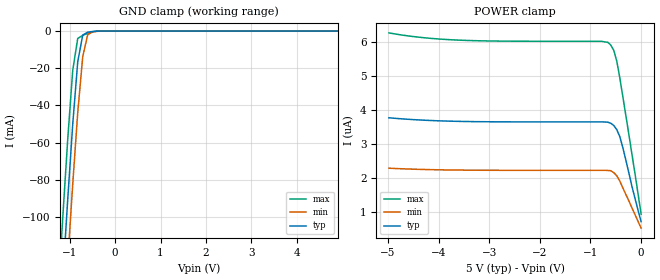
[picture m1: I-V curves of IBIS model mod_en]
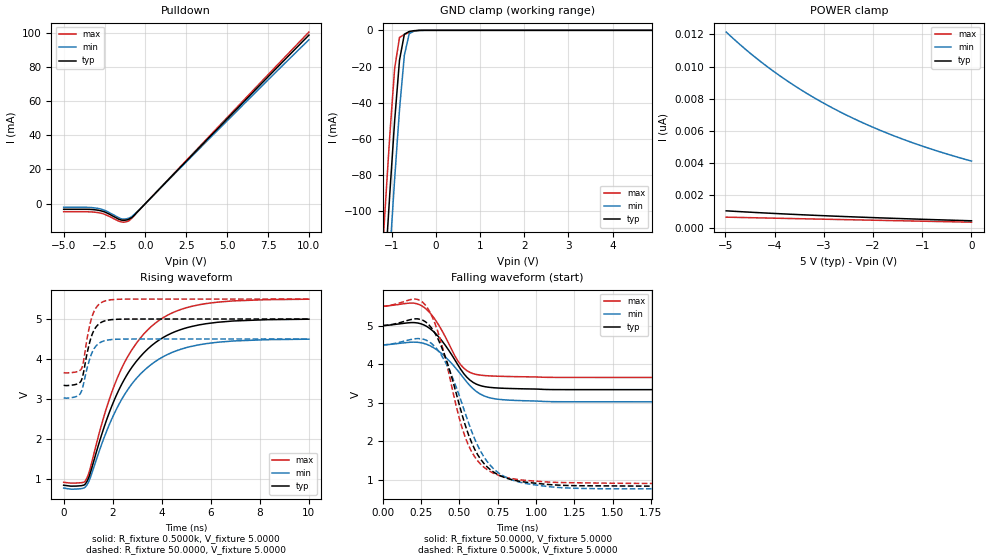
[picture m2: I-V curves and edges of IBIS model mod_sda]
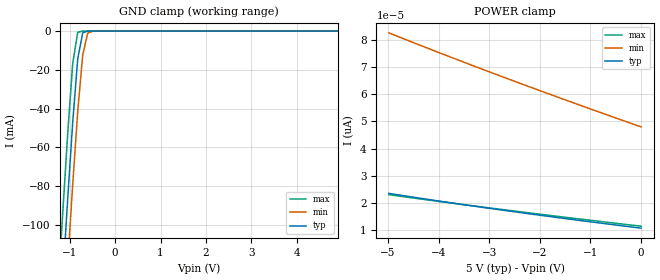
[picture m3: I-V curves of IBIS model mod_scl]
| IBIS (I/O, Buffer, Information, Specification) Model, officially
| electronic behavioral standard for Buffer structures of digital pins.
[IBIS ver]  4.0
[File name] m24c32_fd3_tssop8.ibs
[File Rev]  1.0
[Date]   2 March 2015
[Source]   CAD & Design Services (Catania) - STMicroelectronics
[Notes]
   (Note1)  This IBIS model includes the TSSOP8 package data
   (Note2)  This IBIS model has some Notes about the non-monotonicity
   of the I-V curves, but they are not indicative of problems
   inside the model;
[Copyright] (c) 2015 STMicroelectronics
|   Component M24C32
[Component] M24C32
[Manufacturer] STMicroelectronics
[Package]
| variable   typ   min   max
R_pkg   0.0   0.0   0.0
L_pkg   0.0H   0.0H   0.0H
C_pkg   0.0F   0.0F   0.0F
[Pin]   signal_name   model_name   R_pin   L_pin   C_pin
1   E1   mod_en   NA   NA   NA
2   E2   mod_en   NA   NA   NA
3   E3   mod_en   NA   NA   NA
4   VSS   GND   NA   NA   NA
5   SDA   mod_sda   NA   NA   NA
6   SCL   mod_scl   NA   NA   NA
7   WC   mod_wc   NA   NA   NA
8   VCC   POWER   NA   NA   NA
[Package Model]  182696_TSSOP8
[Define Package Model]  182696_TSSOP8
[Manufacturer]  STMicroelectronics
[OEM]  STMicroelectronics
[Description]  8 pin TSSOP package
[Number Of Pins]  8
[Pin Numbers]
|Pin Num   Terminal Name
1   | net1
2   | net2
3   | net3
4   | net4_GND
5   | net5
6   | net6
7   | net7
8   | net8_VDD
[Model Data]
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[End Model Data]
[End Package Model]
| Models and submodels in the file (4): mod_en (Input), mod_sda (I/O_open_drain), mod_scl (Input), mod_wc (Input)
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|   Model mod_en
[Model]   mod_en
Model_type Input
Vinl   =   1.500V
Vinh   =   3.500V
C_comp   1.763pF   1.683pF   1.933pF
[Temperature Range]   25.0000   85.0000   -40.0000
[Voltage Range]   5.0000V   4.5000V   5.5000V
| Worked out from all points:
|   GND clamp passes 1 mA (typ) near -0.63 V on its own axis
[GND_clamp]
|Voltage   I(typ)   I(min)   I(max)
-5V       -1.778A    -1.809A    -1.75A
-1.26V    -178.1mA   -212mA     -145mA
-1.15V    -133.7mA   -167.6mA   -100.7mA
-1.04V    -90.63mA   -124.1mA   -58.26mA
-930mV    -50.12mA   -82.33mA   -21.13mA
-820mV    -16.52mA   -43.87mA   -3.965mA
-710mV    -2.16mA    -13.76mA   -2.277mA
-600mV    -612.9uA   -1.875mA   -1.25mA
-490mV    -197.3uA   -433.1uA   -365.3uA
-270mV    -576.4nA   -6.871uA   -62.51nA
4.9V      413.9pA    4.479nA    298.2pA
[POWER_clamp]
|Voltage   I(typ)   I(min)   I(max)
-4.98V    3.781uA    2.297uA    6.278uA
-4.32V    3.712uA    2.261uA    6.14uA
-3.6V     3.675uA    2.242uA    6.065uA
-780mV    3.659uA    2.234uA    6.031uA
-660mV    3.651uA    2.231uA    6.002uA
-600mV    3.62uA     2.223uA    5.922uA
-540mV    3.554uA    2.166uA    5.763uA
-480mV    3.429uA    2.073uA    5.439uA
-420mV    3.222uA    1.914uA    4.947uA
-360mV    2.894uA    1.715uA    4.388uA
-180mV    1.752uA    1.124uA    2.692uA
0V        723nA      533.2nA    942nA
|   Model mod_sda
[Model]   mod_sda
Model_type I/O_open_drain
Polarity   Inverting
Vinl   =   1.500V
Vinh   =   3.500V
Vmeas  =   2.500V
Cref   =   10pF
Rref   =   1k
Vref   =   5.000V
C_comp   1.845pF   1.762pF   2.023pF
[Temperature Range]  25.0000   85.0000   -40.0000
[Voltage Range]   5.0000V   4.5000V   5.5000V
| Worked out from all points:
|   slope of the pulldown table from 0 to 0.75 V, typ, clamps not added: 100 ohm
|   GND clamp passes 1 mA (typ) near -0.63 V on its own axis
|   rising waveform, R_fixture 0.5000k, V_fixture 5.0000: 20-80 % time 1.95ns typ, 2ns min, 1.89ns max; typ from 0.836 V to 5 V
|   rising waveform, R_fixture 50.0000, V_fixture 5.0000: 20-80 % time 384ps typ, 405ps min, 365ps max; typ from 3.34 V to 5 V
|   falling waveform, R_fixture 50.0000, V_fixture 5.0000: 20-80 % time 174ps typ, 199ps min, 155ps max; typ from 5 V to 3.34 V
|   falling waveform, R_fixture 0.5000k, V_fixture 5.0000: 20-80 % time 208ps typ, 231ps min, 189ps max; typ from 5 V to 0.836 V
[Pulldown]
|Voltage   I(typ)   I(min)   I(max)
-5V       -3.351mA   -2.158mA   -4.765mA
-3.56V    -3.372mA   -2.214mA   -4.81mA
-2.92V    -3.864mA   -2.805mA   -5.269mA
-2.44V    -5.1mA     -4.182mA   -6.528mA
-1.48V    -9.674mA   -8.935mA   -10.76mA
-1.16V    -9.633mA   -8.945mA   -10.68mA
-1V       -9.127mA   -8.454mA   -10.05mA
-680mV    -6.888mA   -6.316mA   -6.967mA
-360mV    -3.586mA   -3.521mA   -3.635mA
5.4V      53.54mA    52.35mA    54.38mA
10V       98.63mA    95.91mA    100.4mA
[GND_clamp]
|Voltage   I(typ)   I(min)   I(max)
-5V       -1.778A    -1.809A    -1.75A
-1.26V    -178.1mA   -212mA     -145mA
-1.15V    -133.7mA   -167.6mA   -100.7mA
-1.04V    -90.63mA   -124.1mA   -58.26mA
-930mV    -50.12mA   -82.33mA   -21.13mA
-820mV    -16.52mA   -43.87mA   -3.965mA
-710mV    -2.16mA    -13.76mA   -2.277mA
-600mV    -612.9uA   -1.875mA   -1.25mA
-490mV    -197.3uA   -433.1uA   -365.3uA
-270mV    -576.4nA   -6.871uA   -62.51nA
4.9V      413.9pA    4.479nA    298.2pA
[POWER_clamp]
|Voltage   I(typ)   I(min)   I(max)
-4.98V    1.04nA     12.14nA    647.1pA
-4.5V     956.4pA    10.84nA    616pA
-3.96V    870.9pA    9.573nA    581.4pA
-3.42V    793.4pA    8.474nA    547.1pA
-2.82V    715.2pA    7.424nA    509.3pA
-2.16V    637.2pA    6.443nA    468.1pA
-1.5V     566pA      5.61nA     427.2pA
-780mV    494.5pA    4.839nA    382.8pA
0V        422.7pA    4.13nA     334.9pA
[Ramp]
| variable   typ   min   max
dV/dt_r   0.9957/0.4275n   0.8840/0.5215n   1.1057/0.3886n
dV/dt_f   0.9957/0.2040n   0.8841/0.2198n   1.1060/0.1774n
R_load = 50.0000
[Rising Waveform]
R_fixture= 0.5000k
V_fixture= 5.0000
V_fixture_min= 4.5000
V_fixture_max= 5.5000
|time   V(typ)   V(min)   V(max)
0s        836.5mV    764.8mV    909.5mV
880ps     864.6mV    788.9mV    939.7mV
1.05ns    1.075V     965.7mV    1.187V
1.77ns    2.506V     2.218V     2.816V
2.29ns    3.272V     2.904V     3.666V
2.95ns    3.929V     3.502V     4.38V
3.75ns    4.413V     3.941V     4.903V
4.71ns    4.722V     4.229V     5.225V
5.79ns    4.881V     4.381V     5.385V
10ns      4.996V     4.495V     5.496V
[Rising Waveform]
R_fixture= 50.0000
V_fixture= 5.0000
V_fixture_min= 4.5000
V_fixture_max= 5.5000
|time   V(typ)   V(min)   V(max)
0s        3.341V     3.027V     3.657V
500ps     3.363V     3.056V     3.673V
720ps     3.461V     3.182V     3.748V
800ps     3.632V     3.349V     3.91V
940ps     4.096V     3.733V     4.457V
1.04ns    4.364V     3.953V     4.777V
1.18ns    4.643V     4.189V     5.102V
1.4ns     4.856V     4.373V     5.343V
1.7ns     4.957V     4.461V     5.455V
10ns      5V         4.5V       5.5V
[Falling Waveform]
R_fixture= 50.0000
V_fixture= 5.0000
V_fixture_min= 4.5000
V_fixture_max= 5.5000
|time   V(typ)   V(min)   V(max)
0s        5V         4.5V       5.5V
190ps     5.078V     4.571V     5.584V
270ps     5.015V     4.537V     5.472V
370ps     4.686V     4.323V     4.984V
470ps     4.117V     3.929V     4.223V
530ps     3.751V     3.632V     3.895V
610ps     3.486V     3.297V     3.735V
710ps     3.396V     3.121V     3.695V
1.17ns    3.342V     3.028V     3.658V
10ns      3.341V     3.027V     3.657V
[Falling Waveform]
R_fixture= 0.5000k
V_fixture= 5.0000
V_fixture_min= 4.5000
V_fixture_max= 5.5000
|time   V(typ)   V(min)   V(max)
0s        5V         4.5V       5.5V
210ps     5.174V     4.658V     5.687V
280ps     5.096V     4.628V     5.526V
340ps     4.81V      4.457V     5.067V
420ps     4.056V     3.967V     3.965V
500ps     2.945V     3.184V     2.598V
580ps     1.972V     2.267V     1.736V
720ps     1.217V     1.307V     1.183V
900ps     965.2mV    939.8mV    1.006V
10ns      836.5mV    764.8mV    909.5mV
|   Model mod_scl
[Model]   mod_scl
Model_type Input
Vinl   =   1.500V
Vinh   =   3.500V
C_comp   1.763pF   1.683pF   1.933pF
[Temperature Range]   25.0000   85.0000   -40.0000
[Voltage Range]   5.0000V   4.5000V   5.5000V
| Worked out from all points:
|   GND clamp passes 1 mA (typ) near -0.71 V on its own axis
[GND_clamp]
|Voltage   I(typ)   I(min)   I(max)
-5V       -1.733A    -1.764A    -1.703A
-1.26V    -171.7mA   -205.6mA   -137.3mA
-1.15V    -128.4mA   -162.2mA   -94.06mA
-1.04V    -86.41mA   -119.8mA   -52.72mA
-930mV    -46.94mA   -79.03mA   -16.7mA
-820mV    -14.34mA   -41.51mA   -622.7uA
-710mV    -879.9uA   -12.25mA   -4.426uA
-600mV    -18.76uA   -1.026mA   -29.45nA
-490mV    -372.8nA   -42.05uA   -196.9pA
4.9V      10.41pA    50.62pA    10.07pA
[POWER_clamp]
|Voltage   I(typ)   I(min)   I(max)
-4.98V    23.46pA    82.67pA    22.99pA
-3.84V    20.23pA    74.3pA     20.13pA
-2.58V    16.89pA    65.38pA    17.13pA
-1.32V    13.75pA    56.76pA    14.26pA
0V        10.64pA    47.99pA    11.36pA
